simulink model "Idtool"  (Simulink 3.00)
settings: Solver=ode45  SolverMode=SingleTasking  StartTime=0.0  StopTime=10  MaxStep=10  RelTol=1e-3  AbsTol=1e-3
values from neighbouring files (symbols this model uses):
  Au = [a0 a1;a2]    [data_id1.m]    (also in data_id2.m = [a0;[a1 a2]])
  Ay = [A0 A1;A2]    [data_id1.m]    (also in data_id2.m = A0)
  Bu = [b0;b1]    [data_id1.m]    (also in data_id2.m)
  By = [B0;B1]    [data_id1.m]    (also in data_id2.m)
  Cu = [c0 c1]/den(1)    [data_id1.m]    (also in data_id2.m = [c0 c1])
  Cy = [C0;C1]/den(1)    [data_id1.m]    (also in data_id2.m = [C0;C1])
  Du = zeros(in*(cit+1),in)    [data_id1.m]    (also in data_id2.m = zeros(cit*in,in))
  Dy = -[zeros(out,out);By]/den(1)    [data_id1.m]    (also in data_id2.m = [D1;D2])

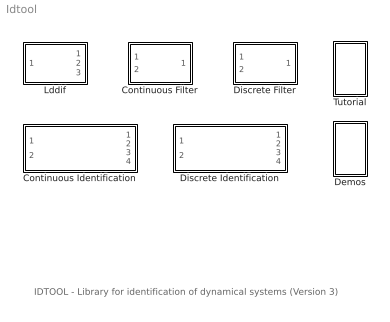
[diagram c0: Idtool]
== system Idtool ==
  note: IDTOOL - Library for identification of dynamical systems (Version 3)
  Continuous Filter : Subsystem  mask(C-Filter){par=[1,1], cit=[0], men=[1], tc=[1]}
      mask prompts: par "No. of inputs and outputs -  [in,out]:"; cit "Numerator degree -  [dn]:"; men "Denominator degree -  [dd]:"; tc "Time constant of the filter - [Tc]:"
      mask help: C-filter: Continuous filters Authors: Lubos Cirka and Miroslav Fikar 1998 - 2004
      mask init:
      | in=par(1); out=par(2);  eval('data_id1');
  Continuous Identification : Subsystem  mask(Continuous Identification){par1=[1,2], tc=[0.5], par2=[0.985,0.01], poc=[0 0 0 0], kov=[10e6], ts=[1]}
      mask prompts: par1 "Degrees of numerator and denominator -  [dn, dd]:"; tc "Time constant of the filter - [Tc]:"; par2 "Exponential forgetting and Bittanti's correction - [L, d]:"; poc "Initial parameter estimates - [theta(1) ... theta(n)]:"; kov "Covariance matrix (see help, standard - [10e6]):"; ts "Sampling time - [ts]:"
      mask help: Continuous identification Authors: Lubos Cirka and Miroslav Fikar 1998 - 2004
      mask init:
      | cit=par1(1);men=par1(2);L=par2(1);d=par2(2); n=cit+men+1;m=1;in=1;out=1;eval('data_id1');
  Demos : Subsystem
  Discrete Filter : Subsystem  mask(D-Filter){par=[1,1], cit=[1], men=[1], ts=[1], Ds=[0]}
      mask prompts: par "No. of inputs and outputs -  [in,out]:"; cit "Numerator degree -  [dn]:"; men "Denominator degree -  [dd]:"; ts "Sampling time - [ts]:"; Ds "Discrete time delay - [D]:"
      mask help: D-filter: Discrete filter Authors: Lubos Cirka and Miroslav Fikar 1998 - 2004
      mask init:
      | in=par(1); out=par(2);  eval('data_id2');
  Discrete Identification : Subsystem  mask(Discrete Identification){par1=[2,2], Ds=[0], par2=[0.985,0.01], poc=[0 0 0 0], kov=[10e6], ts=[1]}
      mask prompts: par1 "Degrees of numerator and denominator -  [dn, dd]:"; Ds "Discrete time delay - [D]:"; par2 "Exponential forgetting and Bittanti's correction - [L, d]:"; poc "Initial parameter estimates - [theta(1) ... theta(n)]:"; kov "Covariance matrix (see help, standard - [10e6]):"; ts "Sampling time - [ts]:"
      mask help: Discrete identification Authors: Lubos Cirka and Miroslav Fikar 1998 - 2004
      mask init:
      | cit=par1(1);men=par1(2);L=par2(1);d=par2(2);n=cit+men;m=1;in=1;out=1;eval('data_id2');
  Lddif : Subsystem  mask(LDDIF){par=[4,1], L=[0.985], d=[0.01], poc=[0 0 0 0], kov=[10e6], ts=[1]}
      mask prompts: par "No. of estimated parameters and outputs - [n,m]:"; L "Exponential forgetting - [L]:"; d "Bittanti's correction - [d]:"; poc "Initial parameter estimates - [theta(1) ... theta(n)]:"; kov "Covariance matrix (see help, standard - [10e6]):"; ts "Sampling period - [ts]:"
      mask help: LDDIF: + Bittanti's corrections Authors: Lubos Cirka and Miroslav Fikar 1998 - 2004
      mask init:
      | n=par(1); m=par(2);
  Tutorial : Subsystem

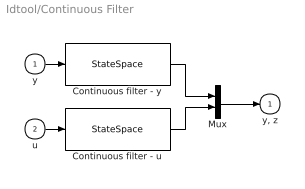
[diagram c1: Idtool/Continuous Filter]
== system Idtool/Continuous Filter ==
  y : Inport  Port=1  PortWidth=-1  SampleTime=-1  DataType=auto
  u : Inport  Port=2  PortWidth=-1  SampleTime=-1  DataType=auto
  Continuous filter - u : StateSpace  A=Au  B=Bu  C=Cu  D=Du  X0=0
  Continuous filter - y : StateSpace  A=Ay  B=By  C=Cy  D=Dy  X0=0
  Mux : Mux  Inputs=2
  "y, z" : Outport  Port=1  InitialOutput=0
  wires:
  Mux/1 -> "y, z"/1
  Continuous filter - u/1 -> Mux/2
  Continuous filter - y/1 -> Mux/1
  u/1 -> Continuous filter - u/1
  y/1 -> Continuous filter - y/1

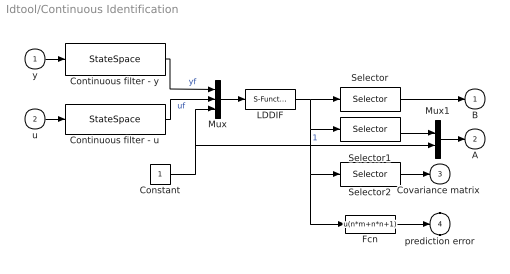
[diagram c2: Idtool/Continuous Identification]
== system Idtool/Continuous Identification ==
  y : Inport  Port=1  PortWidth=-1  SampleTime=-1  DataType=auto
  u : Inport  Port=2  PortWidth=-1  SampleTime=-1  DataType=auto
  Constant : Constant  Value=1
  Continuous filter - u : StateSpace  A=Au  B=Bu  C=Cu  D=Du  X0=0
  Continuous filter - y : StateSpace  A=Ay  B=By  C=Cy  D=Dy  X0=0
  Fcn : Fcn  Expr=u(n*m+n*n+1)
  LDDIF : S-Function  FunctionName=lddif_s  Parameters=m ,n+1 ,L ,d, [poc 0], kov, ts  PortCounts=[]  SFunctionModules=''
  Mux : Mux  Inputs=3
  Mux1 : Mux  Inputs=2
  Selector : Selector  Elements=[men+cit+1:-1:men+1]  InputPortWidth=(n+1)*m+(n+1)*(n+1)+m
  Selector1 : Selector  Elements=[men:-1:1]  InputPortWidth=(n+1)*m+(n+1)*(n+1)+m
  Selector2 : Selector  Elements=[(n+1)*m+1:1:(n+1)*m+(n+1)*(n+1)]  InputPortWidth=(n+1)*m+(n+1)*(n+1)+m
  B : Outport  Port=1  InitialOutput=0
  A : Outport  Port=2  InitialOutput=0
  "Covariance matrix " : Outport  Port=3  InitialOutput=0
  prediction error : Outport  Port=4  InitialOutput=0
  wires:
  LDDIF/1 -> Selector/1, Selector1/1, Selector2/1, Fcn/1
  Continuous filter - u/1 -> Mux/2  "uf"
  Continuous filter - y/1 -> Mux/1  "yf"
  u/1 -> Continuous filter - u/1
  y/1 -> Continuous filter - y/1
  Selector/1 -> B/1
  Mux/1 -> LDDIF/1
  Constant/1 -> Mux/3, Mux1/2  "1"
  Selector1/1 -> Mux1/1
  Mux1/1 -> A/1
  Selector2/1 -> "Covariance matrix "/1
  Fcn/1 -> prediction error/1

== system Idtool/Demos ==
  note: Library of demo blocks

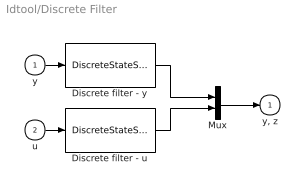
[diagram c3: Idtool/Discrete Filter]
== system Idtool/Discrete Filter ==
  y : Inport  Port=1  PortWidth=-1  SampleTime=-1  DataType=auto
  u : Inport  Port=2  PortWidth=-1  SampleTime=-1  DataType=auto
  Discrete filter - u : DiscreteStateSpace  A=Au  B=Bu  C=Cu  D=Du  X0=0  SampleTime=ts
  Discrete filter - y : DiscreteStateSpace  A=Ay  B=By  C=Cy  D=Dy  X0=0  SampleTime=ts
  Mux : Mux  Inputs=2
  "y, z" : Outport  Port=1  InitialOutput=0
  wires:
  Mux/1 -> "y, z"/1
  Discrete filter - u/1 -> Mux/2
  Discrete filter - y/1 -> Mux/1
  u/1 -> Discrete filter - u/1
  y/1 -> Discrete filter - y/1

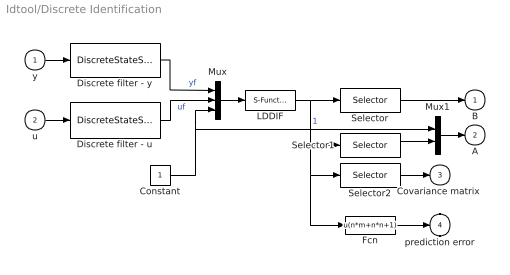
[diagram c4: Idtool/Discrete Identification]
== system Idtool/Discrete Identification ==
  y : Inport  Port=1  PortWidth=-1  SampleTime=-1  DataType=auto
  u : Inport  Port=2  PortWidth=-1  SampleTime=-1  DataType=auto
  Constant : Constant  Value=1
  Discrete filter - u : DiscreteStateSpace  A=Au  B=Bu  C=Cu  D=Du  X0=0  SampleTime=ts
  Discrete filter - y : DiscreteStateSpace  A=Ay  B=By  C=Cy  D=Dy  X0=0  SampleTime=ts
  Fcn : Fcn  Expr=u(n*m+n*n+1)
  LDDIF : S-Function  FunctionName=lddif_s  Parameters=m ,n+1 ,L ,d, [poc 0], kov, ts  PortCounts=[]  SFunctionModules=''
  Mux : Mux  Inputs=3
  Mux1 : Mux  Inputs=2
  Selector : Selector  Elements=[men+1:1:men+cit]  InputPortWidth=(n+1)*m+(n+1)*(n+1)+m
  Selector1 : Selector  Elements=[1:1:men]  InputPortWidth=(n+1)*m+(n+1)*(n+1)+m
  Selector2 : Selector  Elements=[(n+1)*m+1:1:(n+1)*m+(n+1)*(n+1)]  InputPortWidth=(n+1)*m+(n+1)*(n+1)+m
  B : Outport  Port=1  InitialOutput=0
  A : Outport  Port=2  InitialOutput=0
  "Covariance matrix " : Outport  Port=3  InitialOutput=0
  prediction error : Outport  Port=4  InitialOutput=0
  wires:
  Constant/1 -> Mux1/1, Mux/3  "1"
  Selector1/1 -> Mux1/2
  Fcn/1 -> prediction error/1
  Selector2/1 -> "Covariance matrix "/1
  Mux1/1 -> A/1
  Mux/1 -> LDDIF/1
  Selector/1 -> B/1
  y/1 -> Discrete filter - y/1
  u/1 -> Discrete filter - u/1
  Discrete filter - y/1 -> Mux/1  "yf"
  Discrete filter - u/1 -> Mux/2  "uf"
  LDDIF/1 -> Selector/1, Selector1/1, Selector2/1, Fcn/1

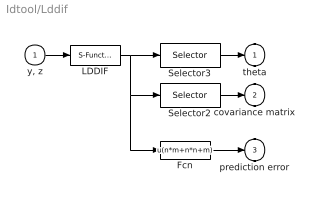
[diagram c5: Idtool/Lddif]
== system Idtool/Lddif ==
  "y, z" : Inport  Port=1  PortWidth=-1  SampleTime=-1  DataType=auto
  Fcn : Fcn  Expr=u(n*m+n*n+m)
  LDDIF : S-Function  FunctionName=lddif_s  Parameters=m, n, L, d, poc, kov, ts  PortCounts=[]  SFunctionModules=''
  Selector2 : Selector  Elements=[n*m:1:n*m+n*n]  InputPortWidth=n*m+n*n+m
  Selector3 : Selector  Elements=[1:1:n*m]  InputPortWidth=n*m+n*n+m
  theta : Outport  Port=1  InitialOutput=0
  covariance matrix : Outport  Port=2  InitialOutput=0
  prediction error : Outport  Port=3  InitialOutput=0
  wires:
  "y, z"/1 -> LDDIF/1
  LDDIF/1 -> Selector3/1, Selector2/1, Fcn/1
  Selector2/1 -> covariance matrix/1
  Selector3/1 -> theta/1
  Fcn/1 -> prediction error/1

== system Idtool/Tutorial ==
  note: Simulations used in tutorial for continuous time identification Simulations used in tutorial for discrete time identification
